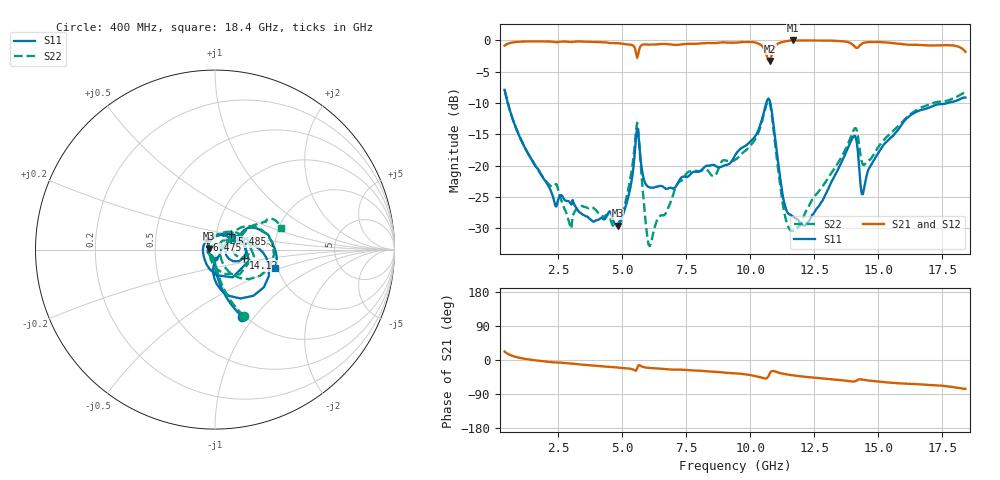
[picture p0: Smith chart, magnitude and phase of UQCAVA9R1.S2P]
!  Part Number  UQCAVA9R1
!  Description: RF capacitor  Mounting Orientation: Horizontal
!  Application:
# GHZ S DB R 50
! Freq  |S11|  S11 Ph  |S21|  S21 Ph  |S12|  S12 Ph  |S22|  S22 Ph
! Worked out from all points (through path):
!   401 points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, 400 MHz to 18.4 GHz, reference 50 ohm
!   highest |S21| = 0.00 dB at 11.65 GHz (marker M1); lowest = -3.3 dB at 10.75 GHz (marker M2)
!   group delay of S21, straight-line fit = 11.6 ps
!   lowest |S11| = -29.6 dB at 4.81 GHz (marker M3), VSWR 1.07, Z = 46.8 + j0.482 ohm
!   |S11| at or under -10 dB: 526 MHz to 10.62 GHz (10.1 GHz wide, 181 % of centre); 10.78 GHz to 17.68 GHz (6.9 GHz wide, 48.5 % of centre)
!   |S22| runs from -32.8 to -7.9 dB; largest |S21 - S12| = 0.0017
!   S11 on the Smith chart (normalised r, x): 400 MHz: 0.97, -0.87; 5.485 GHz: 1.18, +0.21; 6.475 GHz: 0.91, +0.10; 14.12 GHz: 1.37, -0.13; 18.4 GHz: 1.94, -0.45
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0.4  -7.89 -67.9  -0.82 22.1  -0.82 22.1  -7.88 -66.4
1.255  -17.60 -86.2  -0.16 2.4  -0.15 2.4  -17.59 -83.0
2.335  -25.60 -91.2  -0.23 -6.4  -0.23 -6.4  -23.18 -87.6
2.92  -25.70 -92.6  -0.23 -9.4  -0.22 -9.4  -29.06 -102.4
3.415  -27.67 -107.1  -0.18 -12.1  -0.17 -12.2  -26.38 -102.4
4.81  -29.57 171.1  -0.42 -19.8  -0.42 -19.9  -29.45 179.7
5.485  -17.95 43.5  -1.18 -27.5  -1.18 -27.5  -16.63 42.3
5.62  -14.75 -57.5  -2.21 -14.3  -2.21 -14.3  -14.20 -44.9
6.025  -23.39 -172.9  -0.66 -20.9  -0.65 -20.9  -32.62 163.4
6.43  -23.24 134.9  -0.59 -22.5  -0.59 -22.5  -28.17 54.4
6.475  -23.21 130.1  -0.58 -22.7  -0.57 -22.7  -27.99 50.7
7.555  -21.73 74.4  -0.53 -26.6  -0.53 -26.7  -21.02 35.1
9.4  -18.36 34.6  -0.36 -35.3  -0.36 -35.3  -19.03 41.3
10.435  -12.85 4.4  -0.80 -46.5  -0.80 -46.5  -13.21 36.6
10.75  -9.51 -50.3  -3.28 -36.8  -3.28 -36.8  -9.92 -17.6
11.29  -25.29 -83.2  -0.20 -36.4  -0.20 -36.4  -26.69 -47.9
11.65  -28.07 -46.2  0.00 -40.4  0.00 -40.4  -30.36 0.3
12.415  -27.83 5.6  -0.01 -45.9  -0.01 -46.0  -25.39 37.3
14.125  -15.56 -16.4  -1.16 -55.2  -1.16 -55.3  -14.00 -0.6
14.395  -24.54 3.4  -0.43 -51.8  -0.43 -51.9  -19.83 -3.2
15.43  -15.72 31.2  -0.37 -59.7  -0.37 -59.7  -14.96 29.6
18.4  -9.11 -16.9  -1.81 -76.1  -1.81 -76.2  -8.20 18.4
